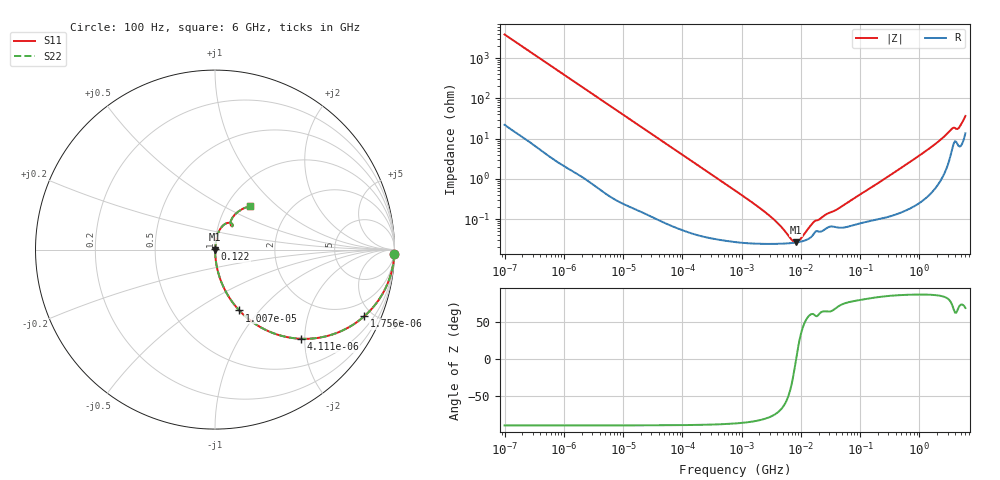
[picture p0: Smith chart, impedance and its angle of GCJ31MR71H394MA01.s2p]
!Murata Part Number: GCJ31MR71H394MA01
!These Parameters are Measured in Series Mode Connection
!Data Generated on Mar 13, 2026
!  o--ll--o
!Port1  Port2
!  o------o
!Operation Temp=25[degC], DC Bias Voltage=0[V]
!Freq. Start=100[Hz] Stop=6[GHz] 401[Steps]
# Hz S RI R 50
!Freq.(Hz) S11(Real) S11(Imag) S21(Real) S21(Imag) S12(Real) S12(Imag) S22(Real) S22(Imag)
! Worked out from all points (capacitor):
!   401 points, 100 Hz to 6 GHz, reference 50 ohm
!   read as one part in series: C = 408 nF near 109 Hz
!   lowest |Z| = 26.4 mohm at 8.312 MHz (marker M1)
!   series resonance near 8.357 MHz, so ESL is about 890 pH
!   S11 on the Smith chart (normalised r, x): 100 Hz: 1, -78; 1.756 kHz: 1.03, -4.48; 4.111 kHz: 1.01, -1.92; 10.07 kHz: 1.00, -0.79; 122 MHz: 1.00, +0.01; 6 GHz: 1.27, +0.68
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100  0.9992 -0.0256  0.000804 0.0256  0.000804 0.0256  0.9992 -0.0256
501  0.9833 -0.1257  0.0167 0.1257  0.0167 0.1257  0.9833 -0.1257
1026  0.9349 -0.244  0.0651 0.244  0.0651 0.244  0.9349 -0.244
1756  0.8324 -0.3706  0.1676 0.3706  0.1676 0.3706  0.8324 -0.3706
2008  0.7921 -0.403  0.2079 0.403  0.2079 0.403  0.7921 -0.403
4111  0.4797 -0.4968  0.5203 0.4968  0.5203 0.4968  0.4797 -0.4968
10066  0.1353 -0.339  0.8647 0.339  0.8647 0.339  0.1353 -0.339
18016  0.0476 -0.2092  0.9524 0.2092  0.9524 0.2092  0.0476 -0.2092
40335  0.0105 -0.0975  0.9895 0.0975  0.9895 0.0975  0.0105 -0.0975
774597  0.000297 -0.00517  0.9997 0.00517  0.9997 0.00517  0.000297 -0.00517
2967816  0.000244 -0.00119  0.9998 0.00119  0.9998 0.00119  0.000244 -0.00119
4440638  0.000246 -0.000656  0.9998 0.000656  0.9998 0.000656  0.000246 -0.000656
7266822  0.000257 -0.000137  0.9997 0.000137  0.9997 0.000137  0.000257 -0.000137
8311524  0.000264 -5.2e-06  0.9997 5.2e-06  0.9997 5.2e-06  0.000264 -5.2e-06
9941735  0.000276 0.000172  0.9997 -0.000172  0.9997 -0.000172  0.000276 0.000172
1.555665e7  0.000384 0.00067  0.9996 -0.00067  0.9996 -0.00067  0.000384 0.00067
1.220122e8  0.000869 0.00485  0.9991 -0.00485  0.9991 -0.00485  0.000869 0.00485
3.124326e8  0.00131 0.012  0.9987 -0.012  0.9987 -0.012  0.00131 0.012
2.450438e9  0.0208 0.0992  0.9792 -0.0992  0.9792 -0.0992  0.0208 0.0992
3.505958e9  0.0693 0.1486  0.9307 -0.1486  0.9307 -0.1486  0.0693 0.1486
4.586474e9  0.0857 0.1455  0.9143 -0.1455  0.9143 -0.1455  0.0857 0.1455
6e9  0.1928 0.2423  0.8072 -0.2423  0.8072 -0.2423  0.1928 0.2423
